// ***************************************************************************
// UDT984

// Datum	  Name	Aktion
// ---------------------------------------------------------------------------
// 29.10.97   Mahler	Neu

TYPE "XC_INIT_SR_UDT"	// User-Auftrag fuer Send/Receive Schnittstelle

STRUCT
	//Aktuelle Werte
	boS5			: BOOL;				//Partner ist S5
	boS7			: BOOL;				//Partner ist S7
      boSEPU		: BOOL;				//Sendepuffer mit Daten belegt
	boREPU		: BOOL;				//Empfangspuffer mit Daten belegt
      boQuitt		: BOOL;				//Warten auf Quittung vom Partner
	res5			: BOOL;
	boINIT		: BOOL;				//Autom. Vorbesetzung ausfuehren
      boError		: BOOL;                       //Sammelfehler

	bPCU			: BYTE;				//Partner PCU-Nummer 0 .. 200
	iID			: INT	;				//ID-Adresse aus Hardwarekonfig.
	wLADDR		: WORD ;				//LADDR aus Hardwarekonfig.

	//Normale Verbindung
	boAS5			: BOOL;				//Partner ist S5
	boAS7			: BOOL;				//Partner ist S7
      boAres2		: BOOL;
      boAres3		: BOOL;
      boAres4		: BOOL;
      boAres5		: BOOL;
      boAres6		: BOOL;
      boAAktiv		: BOOL;				//Kopplung erfolgt ueber diese Schnittstelle

	bAPCU			: BYTE;				//Partner PCU-Nummer 0 .. 200
	iAID			: INT	;				//ID-Adresse aus Hardwarekonfig.
	wALADDR		: WORD ;				//LADDR aus Hardwarekonfig.

	//Reserve Verbindung
	boRS5			: BOOL;				//Partner ist S5
	boRS7			: BOOL;				//Partner ist S7
      boRres2		: BOOL;
      boRres3		: BOOL;
      boRres4		: BOOL;
      boRres5		: BOOL;
      boRres6		: BOOL;
      boRAktiv		: BOOL;                       //Kopplung erfolgt ueber diese Schnittstelle
	bRPCU			: BYTE;				//Partner PCU-Nummer 0 .. 200
	iRID			: INT	;				//ID-Adresse aus Hardwarekonfig.
	wRLADDR		: WORD ;				//LADDR aus Hardwarekonfig.

      //Puffer
	iSendDB		: INT		:= 986;		//DB-Nummer des Sendepuffers
      iSendDW		: INT		:= 0;			//DW-Nummer des Sendepuffers
	iRecvDB		: INT		:= 987;		//DB-Nummer des Empfangspuffers
      iRecvDW		: INT		:= 0;			//DW-Nummer des Empfangspuffers
 	iLEN			: INT		:= 240;		//Laenge 240 Bytes
	bRecvCount		: BYTE;				//Empfangszaehler
	bSendCount		: BYTE;				//Sendezaehler

	//Status Senden
	boSendDONE			:BOOL;
	boSendERROR			:BOOL;
	wSendSTATUS			:WORD;

	//Status Empfangen
	boRecvNDR			:BOOL;
	boRecvERROR			:BOOL;
	wRecvSTATUS			:WORD;
	iRecvLEN			:INT;

	//Verwaltung
	bStep				:BYTE;			//Schrittkette
	bCount1			:BYTE;			//Zaehler Warten auf Senden fertig
	bCount2			:BYTE;			//Zaehler Umschaltung Normal/Reserve

	iPtrJob			:INT;				//Zeiger auf Job fuer Suchen
      iPtrJobSeek			:INT;				//Zeiger suchen

	aRES				:INT;

//Struktur is 50 Bytes lang

END_STRUCT ;

END_TYPE


